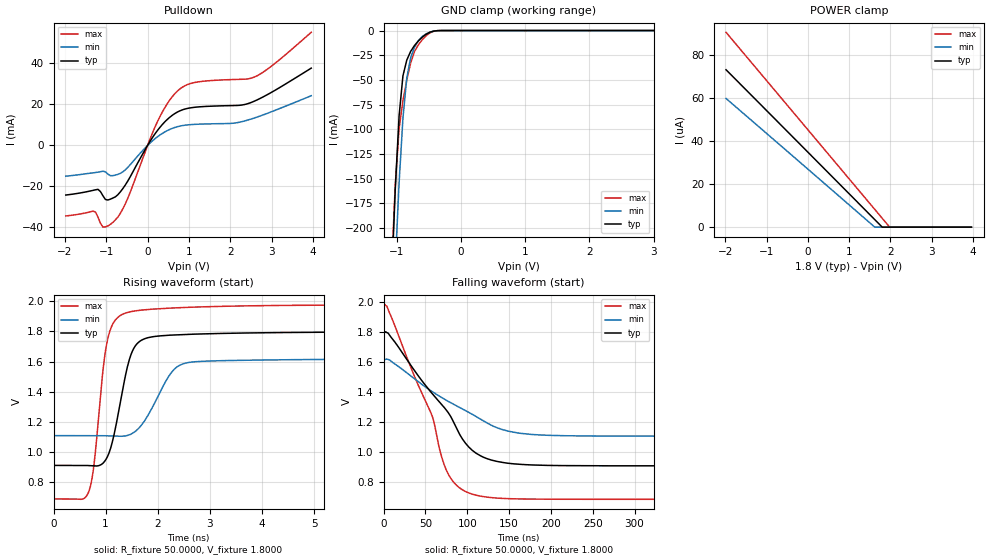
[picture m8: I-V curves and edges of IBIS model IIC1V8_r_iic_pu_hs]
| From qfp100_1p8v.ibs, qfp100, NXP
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[Model] IIC1V8_r_iic_pu_hs
|   Model IIC1V8_r_iic_pu_hs
| This model was characterised for following simulation conditions:
| External (pad) voltage:
|   - Typ: 1.8V,   - Min: 1.62V,   - Max: 1.98V
| Library cells for typ/min/max conditions are connected as defined below:
|  IO - External Pad
|  A - Core Input
|  EN - Output Buffer Enable
|  BOOST - vdde
|  ECS - vdd
|  EGP - gnd
|  ENZI - vdd
|  EPD - vdd
|  EPUN - gnd
|  SSEL - vdd
|  ZI - NC
|  ZIF - NC
|  gnd - gnd
|  gnde - gnde
|  vdd - vdd
|  vdde - vdde
| All other pins connected to ground
Model_type I/O_open_drain
Polarity   Non-Inverting
Enable   Active-Low
Vinl =   0.5400V
Vinh =   1.2600V
Vmeas =  0.9000V
Cref =   0.0F
Rref =   1000.000
Vref =   1.8000V
C_comp   3.6136pF   3.4665pF   3.7543pF
|C_comp_pullup   0.9376pF   0.9156pF   0.9440pF
|C_comp_pulldown   2.3254pF   2.4783pF   2.1797pF
[Model Spec]
| variable   typ   min   max
Vinh   0.5400V   0.4860V   0.5940V
Vinl   1.2600V   1.1340V   1.3860V
Vmeas   0.9000V   0.8100V   0.9900V
Vref   1.8000V   1.6200V   1.9800V
Cref   0.0F   0.0F   0.0F
Rref   1.0000k   1.0000k   1.0000k
[Temperature Range]   25.0000   0.1250k   -40.0000
[Voltage Range]   1.8000V   1.6200V   1.9800V
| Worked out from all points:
|   slope of the pulldown table from 0 to 0.27 V, typ, clamps not added: 33.4 ohm
|   GND clamp passes 1 mA (typ) near -0.44 V on its own axis
|   rising waveform, R_fixture 50.0000, V_fixture 1.8000: 20-80 % time 318ps typ, 487ps min, 235ps max; typ from 0.91 V to 1.8 V
|   falling waveform, R_fixture 50.0000, V_fixture 1.8000: 20-80 % time 66.9ns typ, 88.6ns min, 48.9ns max; typ from 1.8 V to 0.91 V
[Pulldown]
|Voltage   I(typ)   I(min)   I(max)
-1.98V    -24.22mA   -15.04mA   -34.42mA
-1.32V    -21.94mA   -13.4mA    -32.06mA
-1.2V     -21.45mA   -13.05mA   -35.06mA
-1.08V    -24.63mA   -12.6mA    -39.9mA
-900mV    -26.23mA   -14.78mA   -38.53mA
-720mV    -24.07mA   -14.13mA   -34.99mA
-540mV    -19.33mA   -11.9mA    -28.53mA
300mV     8.856mA    5.096mA    14.12mA
720mV     16.26mA    9.117mA    26.48mA
1.14V     18.6mA     10.26mA    30.69mA
2.58V     21.55mA    13.34mA    33.32mA
3.96V     37.7mA     24.26mA    55.17mA
[GND_clamp]
|Voltage   I(typ)   I(min)   I(max)
-1.98V    -2.104A    -2.075A    -2.136A
-1.08V    -259.3mA   -333mA     -246.9mA
-1.02V    -161.8mA   -238.7mA   -157.1mA
-960mV    -86.75mA   -154.7mA   -99.47mA
-900mV    -45.96mA   -88.82mA   -71.06mA
-840mV    -29.91mA   -48mA      -50.26mA
-780mV    -21.16mA   -27.65mA   -32.99mA
-720mV    -15.17mA   -16.88mA   -21.27mA
-660mV    -10.57mA   -10.24mA   -14.57mA
-540mV    -3.796mA   -3.405mA   -5.301mA
-300mV    -21.69uA   -40.85uA   -23.15uA
3.96V     0A         0A         0A
[POWER_clamp]
|Voltage   I(typ)   I(min)   I(max)
-1.98V    73.06uA    59.72uA    90.42uA
1.62V     3.484uA    0A         8.225uA
1.8V      0A         0A         4.113uA
1.98V     0A         0A         0A
3.96V     0A         0A         0A
[Ramp]
| variable   typ   min   max
dV/dt_r  0.5332/0.3184n   0.3066/0.4867n   0.7749/0.2353n
dV/dt_f  0.5332/66.8662n   0.3065/88.5913n   0.7749/48.9352n
R_load = 50.0000
[Rising Waveform]
R_fixture= 50.0000
V_fixture= 1.8000
V_fixture_min= 1.6200
V_fixture_max= 1.9800
|time   V(typ)   V(min)   V(max)
0s        910.3mV    1.108V     687.5mV
675.9ps   909mV      1.108V     735.7mV
775ps     906.6mV    1.108V     910.2mV
1.01ns    952mV      1.107V     1.698V
1.277ns   1.319V     1.104V     1.905V
1.482ns   1.642V     1.117V     1.931V
1.776ns   1.755V     1.221V     1.945V
2.54ns    1.78V      1.59V      1.96V
5.895ns   1.796V     1.615V     1.976V
1us       1.799V     1.619V     1.979V
[Falling Waveform]
R_fixture= 50.0000
V_fixture= 1.8000
V_fixture_min= 1.6200
V_fixture_max= 1.9800
|time   V(typ)   V(min)   V(max)
0s        1.799V     1.619V     1.979V
4.136ns   1.799V     1.622V     1.972V
56.48ns   1.403V     1.411V     1.265V
68.95ns   1.322V     1.367V     977.2mV
77.03ns   1.267V     1.341V     858.2mV
94.29ns   1.089V     1.29V      750.6mV
110.7ns   994.3mV    1.239V     714.5mV
147.3ns   929.2mV    1.144V     692.4mV
206.3ns   912.9mV    1.113V     688mV
1us       910.4mV    1.108V     687.5mV
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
